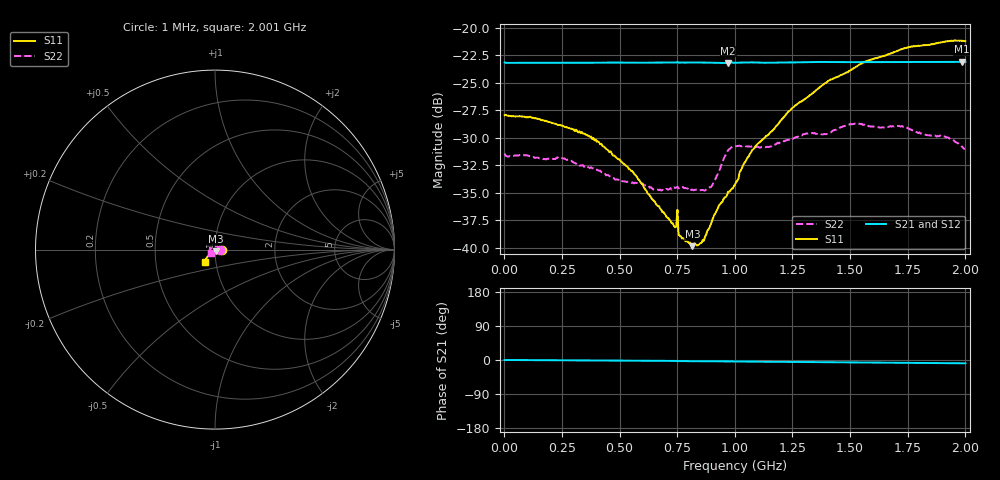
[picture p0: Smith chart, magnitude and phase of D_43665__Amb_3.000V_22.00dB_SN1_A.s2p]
! device id: 43665_
! dir: \\malibu\benchdata\1_engineers\tn_data\43665_75ohm\new\sparar\43665_\amb\3p000v\22p00db
! Serial: 1
! Insertion: A
! Temp: Amb
! VDD: 3.000V
! Attenuation Step: 22.00dB
! IDD: 1.452554e+00mA
! FILE NAME
! DATE 03-27-2009 08:38:45
! CORRECTED  DATA
#  Hz  S  RI  R  75
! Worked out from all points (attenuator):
!   401 points, 1 MHz to 2.001 GHz, reference 75 ohm
!   highest |S21| = -23.09 dB at 1.986 GHz (marker M1); lowest = -23.2 dB at 971 MHz (marker M2)
!   lowest |S11| = -39.9 dB at 816 MHz (marker M3), VSWR 1.02, Z = 75.6 - j1.4 ohm
!   |S11| at or under -10 dB: start of sweep to end of sweep
!   |S22| runs from -34.8 to -28.7 dB; largest |S21 - S12| = 0.00072
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1000000  0.0401 -0.000388  0.0696 -8.51e-05  0.0696 -0.000184  0.0268 -0.000155
2.41e8  0.0362 -0.000723  0.0693 -0.000827  0.0693 -0.000968  0.0224 0.0126
3.36e8  0.0336 -0.00141  0.0694 -0.00123  0.0694 -0.00135  0.0172 0.0163
5.46e8  0.0225 -0.00351  0.0694 -0.00218  0.0694 -0.00244  0.00513 0.0192
6.71e8  0.014 -0.0065  0.0694 -0.00263  0.0694 -0.00293  -0.00275 0.0181
7.36e8  0.0096 -0.0081  0.0695 -0.00297  0.0694 -0.00323  -0.00679 0.0176
7.41e8  0.0094 -0.00807  0.0695 -0.00301  0.0695 -0.00327  -0.00713 0.0173
7.66e8  0.00784 -0.00812  0.0694 -0.00352  0.0694 -0.00344  -0.00888 0.0165
8.16e8  0.00425 -0.00924  0.0694 -0.00385  0.0695 -0.00379  -0.0123 0.0137
8.56e8  0.000912 -0.0105  0.0694 -0.00416  0.0694 -0.00404  -0.0147 0.011
8.96e8  -0.00276 -0.0125  0.0693 -0.00446  0.0693 -0.00429  -0.0171 0.00786
9.71e8  -0.00816 -0.016  0.069 -0.00452  0.0691 -0.00436  -0.027 0.00679
1.001e9  -0.0103 -0.0164  0.0692 -0.00467  0.0693 -0.00443  -0.0279 0.00793
1.086e9  -0.0192 -0.021  0.0694 -0.00547  0.0695 -0.00521  -0.0285 0.00398
1.241e9  -0.0305 -0.0291  0.0693 -0.00611  0.0695 -0.00583  -0.0307 -0.00431
1.336e9  -0.0365 -0.0346  0.0695 -0.00679  0.0697 -0.00645  -0.0321 -0.00888
1.396e9  -0.0406 -0.0389  0.0696 -0.00736  0.0697 -0.00706  -0.0304 -0.0125
1.526e9  -0.0478 -0.0463  0.0693 -0.00806  0.0696 -0.00782  -0.0322 -0.0175
1.671e9  -0.0529 -0.0547  0.0693 -0.00894  0.0695 -0.0087  -0.0295 -0.0199
1.911e9  -0.0571 -0.0649  0.0692 -0.0102  0.0694 -0.00991  -0.0237 -0.0216
1.986e9  -0.0559 -0.067  0.0692 -0.0106  0.0694 -0.0105  -0.0201 -0.0207
2.001e9  -0.0558 -0.0667  0.0692 -0.0106  0.0694 -0.0105  -0.0198 -0.02
